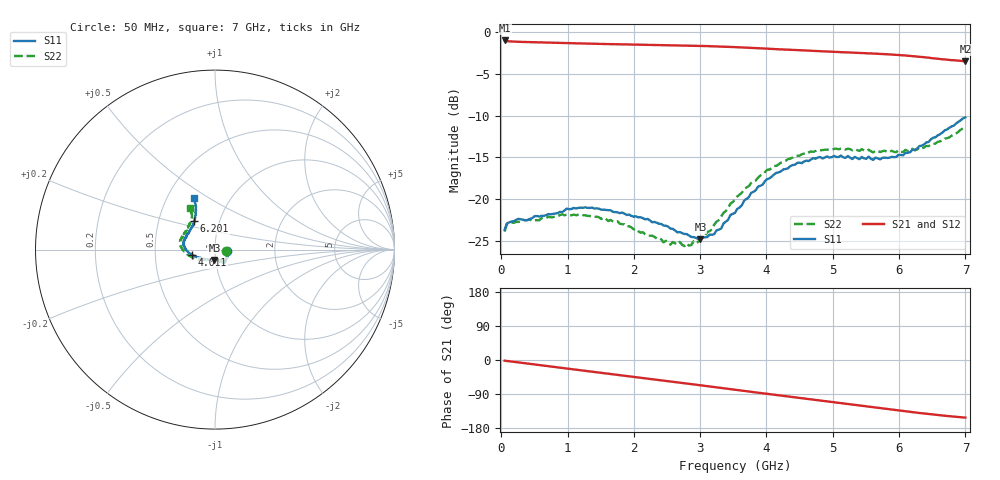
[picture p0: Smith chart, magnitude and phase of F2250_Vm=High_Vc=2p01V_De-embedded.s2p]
! Integrated Device Technology
! Corporate Headquarters
! 6024 Silver Creek Valley Road
! San Jose, CA 95138  USA
! Phone:  1-408-284-8200
! Toll Free:  1-800-223-1366
! Webpage:  http://www.idt.com/
! Timing and RF Division
! 515 Groton Road, Suite 102
! Westford, MA 01886-6024
! Device:  F2250
! Description: Voltage Variable RF Attenuator
! Frequency:  50.0 -  6000.00 MHz
! Package:  3x3 mm Thin QFN Plastic Package: 16 pin
! Ports:  2 RF, 3 DC
!  Pin  1  = GND
!  Pin  2  = NC
!  Pin  3  = RF1  = Port 1
!  Pin  4  = NC
!  Pin  5  = GND
!  Pin  6  = GND
!  Pin  7  = GND
!  Pin  8  = GND
!  Pin  9  = NC
!  Pin 10  = RF2  = Port 2
!  Pin 11  = NC
!  Pin 12  = GND
!  Pin 13  = GND
!  Pin 14  = VCNTRL
!  Pin 15  = VDD
!  Pin 16  = VMODE
! Vcntrl:  2.010 Volts
! Vmode:  +3.300 Volts
! Vdd:  +3.30  Volts
! Current:  1.319 mA
! Data:  The device was measured on a the F2250 evaluation board which has
!  individual transmission lines to the RF pins.  Data was collected
!  using a calibrated network analyzer.  The evaluation board was
!  de-embedded using a TRL calibration technique.
!  The reference plane is the edge of the package pin.
! Misc:  SN 10
!  Action Tracker AT0258
! Date Measured:  2014-11-26
! Date:  2015-10-15  MJV
! Note:
!  Integrated Device Technology supplies this data as a sample of measured
!  data at the package pin for this product.  Your particular data for this
!  product may vary.
!  Data was taken at 25 degrees C.
!  Integrated Device Technology reserves the right to change this data at anytime.
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# GHz S dB R 50
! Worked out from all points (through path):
!   201 points, 50 MHz to 7 GHz, reference 50 ohm
!   highest |S21| = -1.02 dB at 50 MHz (marker M1); lowest = -3.5 dB at 7 GHz (marker M2)
!   group delay of S21, straight-line fit = 61.1 ps
!   lowest |S11| = -24.8 dB at 3.004 GHz (marker M3), VSWR 1.12, Z = 49.4 - j5.69 ohm
!   |S11| at or under -10 dB: start of sweep to end of sweep
!   |S22| runs from -25.6 to -11.4 dB; largest |S21 - S12| = 0.0019
!   S11 on the Smith chart (normalised r, x): 50 MHz: 1.14, -0.02; 4.011 GHz: 0.77, -0.05; 6.201 GHz: 0.75, +0.25; 7 GHz: 0.68, +0.43
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0.05  -23.67 -8.7  -1.02 -1.8  -1.02 -1.8  -23.87 -9.3
0.08475  -22.89 -7.9  -1.10 -2.5  -1.10 -2.5  -23.00 -8.3
0.1195  -22.77 -8.5  -1.13 -3.3  -1.13 -3.2  -22.81 -7.9
0.91875  -21.55 -44.0  -1.32 -21.1  -1.32 -21.1  -21.81 -47.4
1.2315  -21.03 -51.8  -1.39 -27.9  -1.39 -27.9  -21.91 -57.7
1.75275  -21.57 -58.6  -1.48 -39.1  -1.48 -39.1  -22.65 -65.7
2.37825  -22.95 -59.4  -1.57 -52.7  -1.57 -52.8  -24.65 -69.7
2.552  -23.52 -63.6  -1.59 -56.6  -1.59 -56.6  -25.44 -76.2
2.691  -23.93 -70.1  -1.62 -59.7  -1.62 -59.7  -25.10 -83.2
2.7605  -24.16 -72.0  -1.63 -61.2  -1.63 -61.3  -25.62 -87.3
3.00375  -24.79 -93.1  -1.67 -66.7  -1.68 -66.7  -24.64 -108.6
3.21225  -24.17 -114.7  -1.72 -71.4  -1.72 -71.4  -23.02 -126.8
3.525  -21.63 -142.8  -1.82 -78.5  -1.82 -78.5  -20.08 -145.6
3.76825  -19.24 -157.5  -1.91 -84.0  -1.91 -84.0  -18.06 -157.1
4.0115  -17.61 -167.1  -2.01 -89.4  -2.01 -89.4  -16.48 -166.8
4.4285  -15.88 -179.3  -2.17 -98.6  -2.17 -98.6  -14.82 -179.6
4.7065  -15.10 173.3  -2.27 -104.8  -2.27 -104.8  -14.34 174.4
5.054  -14.96 165.0  -2.40 -112.4  -2.39 -112.5  -13.96 167.1
5.85325  -15.04 138.6  -2.69 -129.9  -2.69 -130.0  -14.36 148.1
6.20075  -14.09 126.4  -2.90 -137.6  -2.90 -137.7  -13.97 138.9
6.54825  -12.60 117.8  -3.17 -144.6  -3.17 -144.8  -13.35 127.5
7  -10.22 112.6  -3.50 -152.0  -3.51 -152.1  -11.39 121.1
